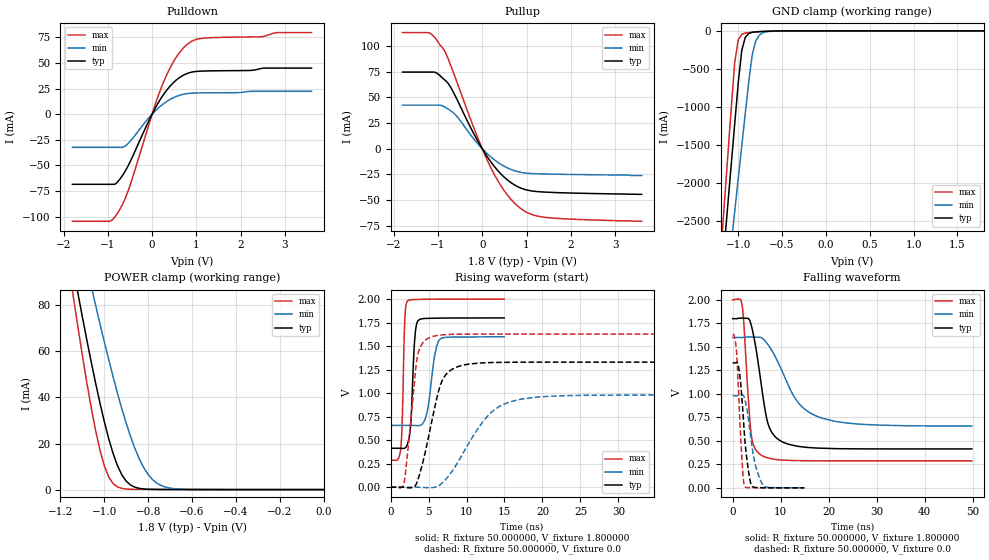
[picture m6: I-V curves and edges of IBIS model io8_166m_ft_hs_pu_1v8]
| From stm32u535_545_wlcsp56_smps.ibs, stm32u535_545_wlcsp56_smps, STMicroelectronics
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|   Model io8_166m_ft_hs_pu_1v8
[Model]  io8_166m_ft_hs_pu_1v8
Model_type I/O
Polarity   Non-Inverting
Enable   Active-Low
Vinl =   0.540000V
Vinh =   1.260000V
Vmeas =  0.900000V
Cref =   50.000000pF
Rref =   100.000000M
Vref =   0.0V
C_comp   3.358200pF   3.352700pF   3.400300pF
[Temperature Range]   25.000000   0.140000k   -40.000000
[Pullup Reference]   1.800000V   1.600000V   2.000000V
[Pulldown Reference]   0.0V   0.0V   0.0V
[POWER Clamp Reference]   1.800000V   1.600000V   2.000000V
[GND Clamp Reference]   0.0V   0.0V   0.0V
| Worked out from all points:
|   slope of the pulldown table from 0 to 0.27 V, typ, clamps not added: 13.6 ohm
|   slope of the pullup table from 0 to 0.27 V, typ, clamps not added: 15.9 ohm
|   GND clamp passes 1 mA (typ) near -0.51 V on its own axis
|   POWER clamp passes 1 mA (typ) near -0.86 V on its own axis
|   rising waveform, R_fixture 50.000000, V_fixture 1.800000: 20-80 % time 469ps typ, 908ps min, 312ps max; typ from 0.414 V to 1.8 V
|   rising waveform, R_fixture 50.000000, V_fixture 0.0: 20-80 % time 2.22ns typ, 4.81ns min, 1.18ns max; typ from 0 V to 1.33 V
|   falling waveform, R_fixture 50.000000, V_fixture 1.800000: 20-80 % time 2.6ns typ, 6.11ns min, 1.3ns max; typ from 1.8 V to 0.414 V
|   falling waveform, R_fixture 50.000000, V_fixture 0.0: 20-80 % time 1.31ns typ, 1.86ns min, 938ps max; typ from 1.33 V to 0 V
[Pulldown]
|Voltage   I(typ)   I(min)   I(max)
-1.8V     -68.38mA   -32.32mA   -104.4mA
-960mV    -68.38mA   -32.32mA   -104.4mA
-780mV    -66.08mA   -32.32mA   -96.43mA
-660mV    -59.2mA    -32.31mA   -87.22mA
-540mV    -50.22mA   -28.51mA   -74.66mA
0V        0A         0A         0A
240mV     18.04mA    9.6mA      29.42mA
480mV     30.68mA    16.02mA    50.95mA
780mV     39.48mA    19.99mA    67.56mA
1.14V     41.99mA    20.78mA    74.01mA
2.82V     44.92mA    22.27mA    79.53mA
3.6V      44.92mA    22.27mA    79.53mA
[Pullup]
|Voltage   I(typ)   I(min)   I(max)
-1.8V     74.47mA    42.39mA    112.9mA
-1.2V     74.47mA    42.39mA    112.8mA
-1.02V    73.36mA    42.39mA    105.2mA
-840mV    66.54mA    40.38mA    94.52mA
-600mV    50.53mA    32.7mA     68.13mA
-180mV    13.77mA    8.913mA    19.32mA
180mV     -11.9mA    -7.442mA   -17.26mA
480mV     -26.98mA   -16.65mA   -39.76mA
840mV     -37.65mA   -22.63mA   -57.07mA
1.08V     -40.74mA   -24.01mA   -63.22mA
1.44V     -42.19mA   -24.58mA   -66.73mA
3.6V      -44.3mA    -26mA      -70.5mA
[GND_clamp]
|Voltage   I(typ)   I(min)   I(max)
-1.8V     -9.908A    -9.683A    -9.994A
-1.2V     -3.383A    -4.084A    -2.934A
-1.16V    -2.841A    -3.655A    -2.294A
-1.12V    -2.299A    -3.226A    -1.656A
-1.04V    -1.218A    -2.369A    -414.2mA
-1V       -684.7mA   -1.941A    -119.2mA
-960mV    -257.2mA   -1.514A    -45.66mA
-920mV    -87.03mA   -1.089A    -28.93mA
-840mV    -19.35mA   -312.8mA   -18.97mA
-800mV    -13.55mA   -132.4mA   -15.49mA
-720mV    -8.042mA   -25.67mA   -9.491mA
1.8V      0A         13.64nA    0A
[POWER_clamp]
|Voltage   I(typ)   I(min)   I(max)
-1.8V     470.9mA    433.7mA    554.6mA
-1.14V    95.28mA    122.7mA    82.88mA
-1.12V    85mA       114mA      70.34mA
-1.06V    55.55mA    88.43mA    35.73mA
-1.04V    46.38mA    80.17mA    25.83mA
-1V       29.54mA    64.14mA    10.37mA
-940mV    10.43mA    41.88mA    1.177mA
-900mV    3.66mA     28.79mA    250.5uA
-840mV    527.2uA    13.26mA    95.94uA
-800mV    154uA      6.55mA     88.4uA
-740mV    59.84uA    1.741mA    70.38uA
0V        0A         18.18nA    0A
[Ramp]
| variable   typ   min   max
dV/dt_r  0.79757/2.21785n   0.58806/4.79425n   0.97651/1.17823n
dV/dt_f  0.83133/2.59825n   0.56527/6.09062n   1.02743/1.29895n
R_load = 50.000000
[Rising Waveform]
R_fixture= 50.000000
V_fixture= 1.800000
V_fixture_min= 1.600000
V_fixture_max= 2.000000
|time   V(typ)   V(min)   V(max)
0s        414.4mV    657.5mV    287.6mV
1.351ns   414mV      657.5mV    420.5mV
1.862ns   415.2mV    657.5mV    1.762V
2.192ns   451.8mV    657.5mV    1.976V
2.673ns   695.6mV    657.4mV    1.993V
3.213ns   1.606V     656.5mV    1.995V
3.634ns   1.772V     655.2mV    1.997V
4.805ns   1.795V     797.5mV    1.999V
6.547ns   1.798V     1.577V     2V
14.95ns   1.8V       1.6V       2V
[Rising Waveform]
R_fixture= 50.000000
V_fixture= 0.0
V_fixture_min= 0.0
V_fixture_max= 0.0
|time   V(typ)   V(min)   V(max)
0s        426.7uV    509.8uV    388.3uV
1.802ns   -699.8uV   507.5uV    56.39mV
3.504ns   58.04mV    522.3uV    1.378V
4.104ns   221.3mV    -1.811mV   1.518V
5.005ns   537.3mV    -4.752mV   1.585V
6.807ns   1.135V     46.3mV     1.62V
9.51ns    1.297V     357.6mV    1.627V
13.31ns   1.326V     799.4mV    1.628V
17.32ns   1.329V     938.6mV    1.628V
49.85ns   1.33V      980.7mV    1.628V
[Falling Waveform]
R_fixture= 50.000000
V_fixture= 1.800000
V_fixture_min= 1.600000
V_fixture_max= 2.000000
|time   V(typ)   V(min)   V(max)
0s        1.8V       1.6V       2V
1.902ns   1.806V     1.6V       1.961V
2.302ns   1.806V     1.601V     1.769V
3.804ns   1.744V     1.605V     596.3mV
5.606ns   1.23V      1.602V     360.8mV
7.608ns   648.1mV    1.507V     315.4mV
11.61ns   464.7mV    1.091V     293mV
14.91ns   434mV      841.6mV    289.1mV
21.32ns   417.9mV    708.4mV    287.8mV
49.85ns   414.4mV    657.5mV    287.6mV
[Falling Waveform]
R_fixture= 50.000000
V_fixture= 0.0
V_fixture_min= 0.0
V_fixture_max= 0.0
|time   V(typ)   V(min)   V(max)
0s        1.33V      980.7mV    1.628V
720.7ps   1.332V     980.7mV    1.499V
1.381ns   1.244V     980.5mV    857.5mV
2.072ns   856.9mV    986.5mV    200.6mV
2.492ns   541.6mV    952.7mV    17.3mV
3.153ns   232.8mV    777.7mV    3.568mV
3.844ns   37.37mV    513mV      2.009mV
4.745ns   4.99mV     241.5mV    1.33mV
6.306ns   1.877mV    32.4mV     901.9uV
14.95ns   426.7uV    509.8uV    388.3uV
